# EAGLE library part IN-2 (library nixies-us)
IN-2: tiny numeric topview nixie tube
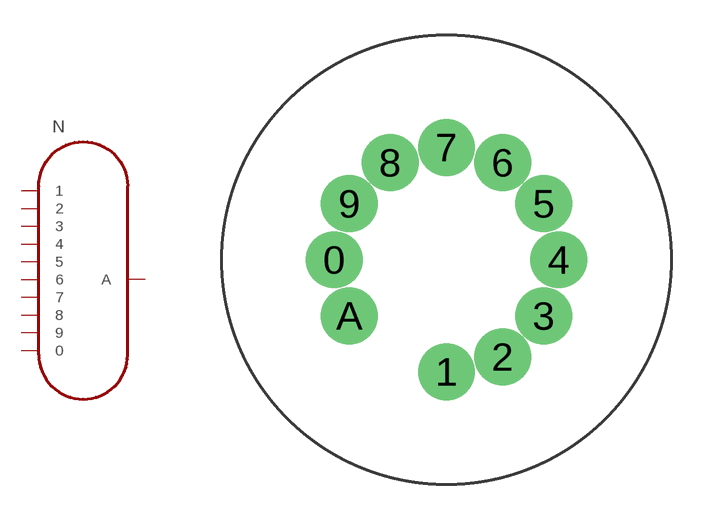
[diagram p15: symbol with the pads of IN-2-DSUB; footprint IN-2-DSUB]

Designator prefix N

## IN-2  [IN-2-DSUB]
0  0
1  1
2  2
3  3
4  4
5  5
6  6
7  7
8  8
9  9
A  A

## Footprint IN-2-DSUB (pad centres in mm)
drill 1.6 pad 2.184: 0 -4.75,0; 1 0,-4.75; 2 2.375,-4.113; 3 4.113,-2.375; 4 4.75,0; 5 4.113,2.375; 6 2.375,4.113; 7 0,4.75; 8 -2.375,4.113; 9 -4.113,2.375; A -4.113,-2.375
